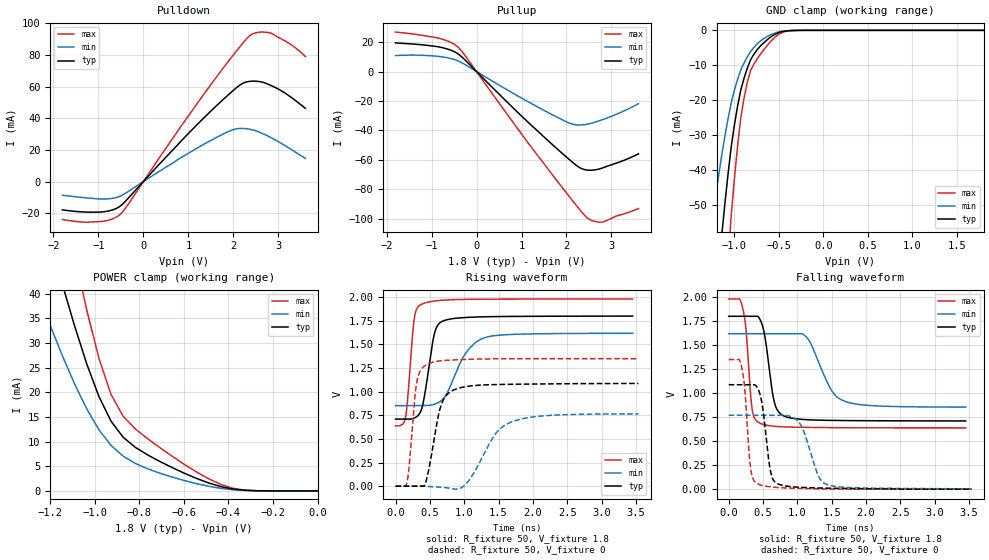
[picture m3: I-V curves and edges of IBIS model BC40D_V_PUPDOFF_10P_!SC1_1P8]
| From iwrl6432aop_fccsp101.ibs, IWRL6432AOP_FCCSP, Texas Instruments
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|   Model Cell BC40D_V_PUPDOFF_10P_!SC1_1P8
|BC40D_V_PUPDOFF_10P_!SC1_1P8
[Model]   BC40D_V_PUPDOFF_10P_!SC1_1P8
Model_type   I/O
Polarity   Non-Inverting
Enable   Active-Low
Vinl =  0.63
Vinh =  1.17
Cref =  15pF
Rref =  100.0000M
Vref =  0V
Vmeas =  0.9
C_comp   2.290246p   2.205796p   2.292736p
|[Input load] weak_pupdoff
|[Output drive] fast
|[supplytol] 10
|[temp] ind
[Model Spec]
Vinl   0.63   0.567   0.693
Vinh   1.17   1.053   1.287
[Temperature Range]   25   125   -40
[Voltage Range]   1.8   1.62   1.98
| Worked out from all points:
|   slope of the pulldown table from 0 to 0.27 V, typ, clamps not added: 32.2 ohm
|   slope of the pullup table from 0 to 0.27 V, typ, clamps not added: 32.5 ohm
|   GND clamp passes 1 mA (typ) near -0.53 V on its own axis
|   POWER clamp passes 1 mA (typ) near -0.44 V on its own axis
|   rising waveform, R_fixture 50, V_fixture 1.8: 20-80 % time 141ps typ, 321ps min, 87.5ps max; typ from 0.709 V to 1.8 V
|   rising waveform, R_fixture 50, V_fixture 0: 20-80 % time 174ps typ, 380ps min, 99ps max; typ from 0 V to 1.09 V
|   falling waveform, R_fixture 50, V_fixture 1.8: 20-80 % time 128ps typ, 290ps min, 84.1ps max; typ from 1.8 V to 0.71 V
|   falling waveform, R_fixture 50, V_fixture 0: 20-80 % time 111ps typ, 211ps min, 81.2ps max; typ from 1.09 V to 0 V
| Nom Voltages:
|   VDD=1.1001, VDDS=1.8, VDDS18=1.8, ESD_BIASFET=0, VSS=0, VSSS=0
| Min Voltages:
|   VDD=0.99, VDDS=1.62, VDDS18=1.62, ESD_BIASFET=0, VSS=0, VSSS=0
| Max Voltages:
|   VDD=1.21, VDDS=1.98, VDDS18=1.98, ESD_BIASFET=0, VSS=0, VSSS=0
[POWER_clamp]
|   voltage   I(typ)   I(min)   I(max)
-1.8V     158.8mA    112.5mA    219.7mA
-1.255V   59.93mA    40mA       84.85mA
-1.127V   39.08mA    25.51mA    55.74mA
-1.055V   28.36mA    18.34mA    40.4mA
-981.8mV  19.18mA    12.43mA    26.97mA
-927.3mV  14.16mA    9.242mA    19.58mA
-872.7mV  10.89mA    7.052mA    15.14mA
-818.2mV  8.843mA    5.581mA    12.58mA
-600mV    3.63mA     2.129mA    5.448mA
-436.4mV  903.9uA    539.1uA    1.358mA
-327.3mV  138.2uA    94.86uA    160.4uA
0V        19.3nA     120.3nA    352.8nA
[Pulldown]
|   voltage   I(typ)   I(min)   I(max)
-1.8V     -17.92mA   -8.674mA   -24.03mA
-927.3mV  -19.22mA   -10.99mA   -25.2mA
-654.5mV  -17.65mA   -10.46mA   -23.22mA
-490.9mV  -14.97mA   -8.904mA   -20.12mA
872.7mV   26.63mA    15.72mA    36.29mA
1.691V    49.7mA     28.87mA    68.59mA
2.127V    60.63mA    33.53mA    84.59mA
2.4V      63.43mA    32.84mA    92.9mA
2.618V    62.99mA    30.74mA    94.47mA
2.836V    60.69mA    27.76mA    93.76mA
3.273V    53.49mA    20.53mA    86.73mA
3.6V      46.26mA    14.64mA    79.11mA
[Pullup]
|   voltage   I(typ)   I(min)   I(max)
-1.8V     19.47mA    10.86mA    26.81mA
-818.2mV  16.61mA    10.18mA    22.5mA
-545.5mV  14.21mA    8.665mA    19.39mA
-381.8mV  11.35mA    6.855mA    15.77mA
1.036V    -31.31mA   -18.66mA   -43.94mA
1.909V    -55.72mA   -32.86mA   -78.99mA
2.182V    -62.87mA   -36.1mA    -89.59mA
2.345V    -66.12mA   -36.26mA   -95.76mA
2.455V    -66.95mA   -35.82mA   -99.33mA
2.618V    -66.9mA    -34.58mA   -101.8mA
2.782V    -65.72mA   -32.89mA   -102.4mA
3.6V      -55.92mA   -21.86mA   -93.15mA
[GND_clamp]
|   voltage   I(typ)   I(min)   I(max)
-1.8V     -270.2mA   -170.2mA   -430.1mA
-1.255V   -91.66mA   -55.91mA   -148.4mA
-1.145V   -59.91mA   -36.44mA   -97.09mA
-1.109V   -50.48mA   -30.83mA   -81.55mA
-1.073V   -41.73mA   -25.65mA   -67.05mA
-1.036V   -33.66mA   -20.92mA   -53.59mA
-927.3mV  -17.07mA   -11.35mA   -25.04mA
-854.5mV  -10.86mA   -7.616mA   -14.91mA
-781.8mV  -6.919mA   -4.945mA   -9.771mA
-636.4mV  -2.823mA   -1.868mA   -4.529mA
-381.8mV  -84.73uA   -78.7uA    -126.1uA
1.8V      19.3nA     3.129uA    310.3nA
[Ramp]
| variable   typ   min   max
dV/dt_f 0.66582244/0.13064135n 0.47095698/0.29741514n 0.81505832/85.878667p
dV/dt_r 0.66457081/0.1768972n 0.48134805/0.39636116n 0.81913391/99.774546p
R_load = 50
[Rising Waveform]
R_fixture = 50
V_fixture = 1.8
V_fixture_min = 1.62
V_fixture_max = 1.98
|   time   V(typ)   V(min)   V(max)
0s        709.4mV    852.1mV    638.8mV
143.7ps   709.4mV    852.1mV    723.5mV
176.4ps   709.4mV    852.1mV    921.3mV
269.4ps   720.7mV    852.1mV    1.755V
369.4ps   795.8mV    852.1mV    1.922V
561.6ps   1.6V       866.3mV    1.959V
688.2ps   1.747V     919.4mV    1.968V
1.012ns   1.785V     1.396V     1.977V
1.287ns   1.792V     1.568V     1.979V
3.453ns   1.8V       1.618V     1.98V
[Rising Waveform]
R_fixture = 50
V_fixture = 0
V_fixture_min = 0
V_fixture_max = 0
|   time   V(typ)   V(min)   V(max)
0s        0V         0V         0V
165.8ps   0V         0V         40.09mV
306.2ps   0V         0V         1.087V
459ps     93.4mV     -2.756mV   1.289V
653.5ps   834.7mV    -10.24mV   1.326V
845.5ps   1.018V     -30.16mV   1.336V
1.044ns   1.056V     37.25mV    1.342V
1.449ns   1.075V     547mV      1.348V
1.676ns   1.078V     676.2mV    1.349V
3.538ns   1.087V     765.1mV    1.35V
[Falling Waveform]
R_fixture = 50
V_fixture = 1.8
V_fixture_min = 1.62
V_fixture_max = 1.98
|   time   V(typ)   V(min)   V(max)
0s        1.8V       1.619V     1.979V
200.1ps   1.8V       1.619V     1.897V
252.3ps   1.8V       1.619V     1.661V
340ps     1.8V       1.619V     840.9mV
445.1ps   1.782V     1.619V     690.7mV
662ps     914.5mV    1.619V     655mV
801.1ps   763.4mV    1.619V     648.7mV
1.144ns   723.3mV    1.575V     643.6mV
1.675ns   714.4mV    919.6mV    639.5mV
3.453ns   710.3mV    854.5mV    638mV
[Falling Waveform]
R_fixture = 50
V_fixture = 0
V_fixture_min = 0
V_fixture_max = 0
|   time   V(typ)   V(min)   V(max)
0s        1.088V     769.9mV    1.35V
185.3ps   1.088V     769.9mV    1.282V
233.6ps   1.088V     769.9mV    1.05V
318.7ps   1.088V     769.9mV    222mV
422.3ps   1.051V     769.9mV    56.06mV
612.7ps   175.3mV    769.9mV    23.54mV
716.8ps   55.1mV     769.9mV    17.03mV
1.032ns   19.58mV    687.3mV    7.824mV
1.43ns    10.46mV    47.83mV    2.07mV
3.538ns   0V         3.566mV    0V
